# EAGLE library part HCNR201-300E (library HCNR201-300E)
Broadcom, HCNR201-300E DC Input Photodiode Output Optocoupler, Surface Mount, 8-Pin PDIP-W Source: Datasheet
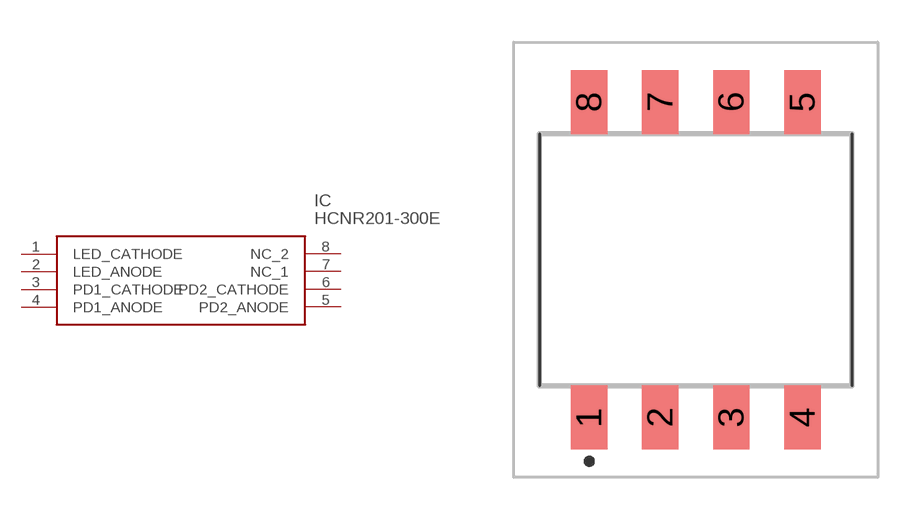
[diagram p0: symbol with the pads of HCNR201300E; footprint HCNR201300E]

Designator prefix IC

## HCNR201-300E (Description: Broadcom, HCNR201-300E DC Input Photodiode Output Optocoupler, Surface Mount, 8-Pin PDIP-W; Height: 5mm; Manufacturer_Name: Avago Technologies; Manufacturer_Part_Number: HCNR201-300E; Mouser_Part_Number: 630-HCNR201-300E; Mouser_Price-Stock: https://www.mouser.co.uk/ProductDetail/Broadcom-Avago/HCNR201-300E?qs=xnajaXqBF9%2Fpqjck28%2FBeQ%3D%3D)  [HCNR201300E]
1  LED_CATHODE
2  LED_ANODE
3  PD1_CATHODE
4  PD1_ANODE
5  PD2_ANODE
6  PD2_CATHODE
7  NC_1
8  NC_2

## Footprint HCNR201300E (pad centres in mm)
HCNR201-300E
smd 1.3 x 2.29: 1 -3.81,-5.635; 2 -1.27,-5.635; 3 1.27,-5.635; 4 3.81,-5.635; 5 3.81,5.635; 6 1.27,5.635; 7 -1.27,5.635; 8 -3.81,5.635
